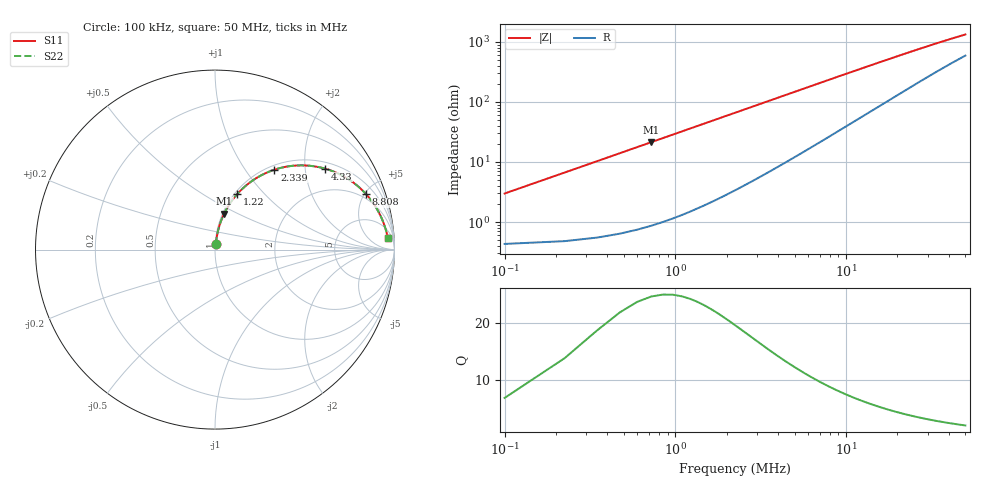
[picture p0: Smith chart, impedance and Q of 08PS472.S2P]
! Coilcraft 0805PS-472 Power Chip Inductor
! 5 February 2003
# MHZ S MA R 50
!Freq  MagS11  AngS11  MagS21  AngS21  MagS12  AngS12  MagS22  AngS22
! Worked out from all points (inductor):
!   403 points, 100 kHz to 50 MHz, reference 50 ohm
!   read as one part in series: L = 4.7 uH near 348.8 kHz
!   highest Q = 24.2 at 722 kHz (marker M1), where L = 4.7 uH
!   S11 on the Smith chart (normalised r, x): 100 kHz: 1.01, +0.06; 1.22 MHz: 1.03, +0.72; 2.339 MHz: 1.07, +1.38; 4.33 MHz: 1.19, +2.55; 8.808 MHz: 1.63, +5.13; 50 MHz: 13, +24
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0.1  0.02971 80.0  0.9953 -1.7  0.9953 -1.7  0.02971 80.0
0.2244  0.06602 82.1  0.9931 -3.8  0.9931 -3.8  0.06602 82.1
0.4732  0.1378 79.5  0.9842 -7.9  0.9842 -7.9  0.1378 79.5
0.5976  0.1728 77.6  0.9777 -9.9  0.9777 -9.9  0.1728 77.6
0.722  0.2071 75.7  0.9699 -11.9  0.9699 -11.9  0.2071 75.7
0.9708  0.273 71.9  0.9511 -15.8  0.9511 -15.8  0.273 71.9
1.2196  0.3348 68.1  0.9286 -19.5  0.9286 -19.5  0.3348 68.1
1.7172  0.4445 61.0  0.8758 -26.4  0.8758 -26.4  0.4445 61.0
2.3392  0.5552 53.3  0.8033 -33.7  0.8033 -33.7  0.5552 53.3
3.21  0.6676 44.7  0.7044 -41.8  0.7044 -41.8  0.6676 44.7
4.3296  0.7604 36.4  0.5954 -49.3  0.5954 -49.3  0.7604 36.4
5.2004  0.8072 31.6  0.5266 -53.5  0.5266 -53.5  0.8072 31.6
6.0712  0.8401 27.9  0.4698 -56.8  0.4698 -56.8  0.8401 27.9
8.4348  0.8916 20.9  0.3599 -62.3  0.3599 -62.3  0.8916 20.9
8.808  0.8968 20.1  0.3468 -62.9  0.3468 -62.9  0.8968 20.1
12.4156  0.9275 14.6  0.2557 -66.4  0.2557 -66.4  0.9275 14.6
16.7696  0.9436 11.0  0.194 -67.7  0.194 -67.7  0.9436 11.0
20.626  0.9508 9.0  0.1602 -67.7  0.1602 -67.7  0.9508 9.0
25.1044  0.9559 7.4  0.1336 -67.1  0.1336 -67.1  0.9559 7.4
33.4392  0.9609 5.6  0.103 -65.0  0.103 -65.0  0.9609 5.6
41.774  0.9637 4.5  0.0848 -62.4  0.0848 -62.4  0.9637 4.5
50  0.9654 3.7  0.07292 -59.8  0.07292 -59.8  0.9654 3.7
